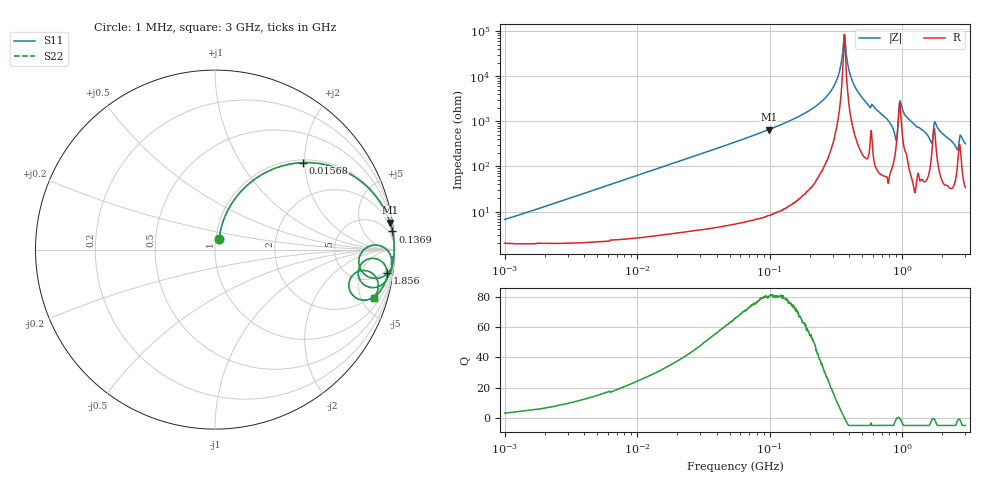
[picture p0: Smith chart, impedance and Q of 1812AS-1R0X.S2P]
!s-Parameter Generated by FASTRON Sdn. Bhd.
!FASTRON P/N : 1812AS-1R0X
!Keysight Technologies,E4991B,MY54100416,A.01.15
!Date created: Fri Oct 13 15:23:31 2023
!Version  : Rev00 Fri Oct 13 15:23:31 2023
!Data & Calibration Information:
!Freq	S11	S21	S12	S22
!PortZ  Port1:50+j0  Port2:50+j0
!When reading, reference impedance value at option line is always used.
! Remarks : This data is being provided solely for informational purposes.
# Hz S dB R 50
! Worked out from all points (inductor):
!   1601 points, 1 MHz to 3 GHz, reference 50 ohm
!   read as one part in series: L = 1.01 uH near 1.041 MHz
!   highest Q = 80.7 at 98.36 MHz (marker M1), where L = 1.06 uH
!   self-resonance near 366.8 MHz
!   S11 on the Smith chart (normalised r, x): 1 MHz: 1.04, +0.13; 15.68 MHz: 1.06, +1.96; 136.9 MHz: 1, +20; 1.856 GHz: 3, -14; 3 GHz: 1.68, -6.31
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1000000  -23.71 69.0  -0.19 -3.6  -0.19 -3.6  -23.71 69.0
3804036  -12.75 71.9  -0.41 -13.3  -0.41 -13.3  -12.75 71.9
1.447069e7  -3.60 46.8  -2.74 -41.3  -2.74 -41.3  -3.60 46.8
1.567691e7  -3.23 44.7  -3.06 -43.6  -3.06 -43.6  -3.23 44.7
5.477226e7  -0.38 16.0  -11.17 -73.1  -11.17 -73.1  -0.38 16.0
9.836149e7  -0.12 8.7  -16.41 -80.6  -16.41 -80.6  -0.12 8.7
1.368536e8  -0.06 5.8  -19.85 -83.4  -19.85 -83.4  -0.06 5.8
2.083556e8  -0.02 3.0  -25.50 -85.9  -25.50 -85.9  -0.02 3.0
3.062963e8  -0.01 0.9  -35.75 -85.3  -35.75 -85.3  -0.01 0.9
3.334925e8  -0.01 0.5  -41.25 -82.1  -41.25 -82.1  -0.01 0.5
3.667557e8  -0.01 0.0  -58.49 -0.7  -58.49 -0.7  -0.01 0.0
4.0536e8  -0.01 -0.5  -40.61 81.6  -40.61 81.6  -0.01 -0.5
4.548043e8  -0.01 -1.2  -33.84 84.6  -33.84 84.6  -0.01 -1.2
7.925923e8  -0.08 -5.7  -20.03 81.6  -20.03 81.6  -0.08 -5.7
8.892696e8  -1.02 -10.3  -13.88 51.9  -13.88 51.9  -1.02 -10.3
9.828732e8  -0.17 -2.1  -27.65 60.6  -27.65 60.6  -0.17 -2.1
1.621129e9  -0.73 -13.2  -12.57 63.5  -12.57 63.5  -0.73 -13.2
1.773925e9  -0.47 -5.0  -20.00 55.9  -20.00 55.9  -0.47 -5.0
1.855641e9  -0.28 -7.7  -17.31 72.5  -17.31 72.5  -0.28 -7.7
2.530652e9  -1.02 -18.4  -9.85 60.9  -9.85 60.9  -1.02 -18.4
2.783064e9  -0.73 -10.6  -14.24 60.3  -14.24 60.3  -0.73 -10.6
3e9  -0.67 -16.9  -10.70 67.0  -10.70 67.0  -0.67 -16.9
